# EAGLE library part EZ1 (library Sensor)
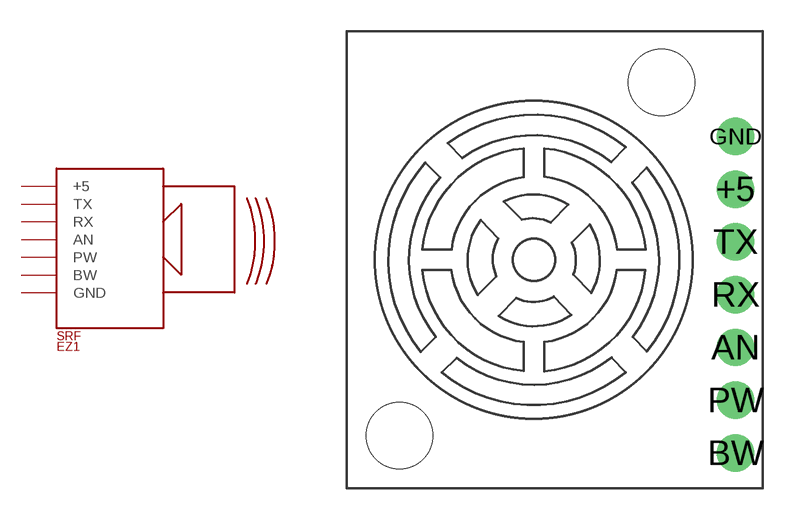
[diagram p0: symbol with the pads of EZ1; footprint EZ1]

Designator prefix SRF

## EZ1  [EZ1]
+5  +5
AN  AN
BW  BW
GND  GND
PW  PW
RX  RX
TX  TX

## Footprint EZ1 (pad centres in mm)
drill 1.2: +5 8.7,3.4; AN 8.7,-4.22; BW 8.7,-9.3; GND 8.7,5.94; PW 8.7,-6.76; RX 8.7,-1.68; TX 8.7,0.86
hole 3.2 at 5.14,8.54
hole 3.2 at -7.46,-8.46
